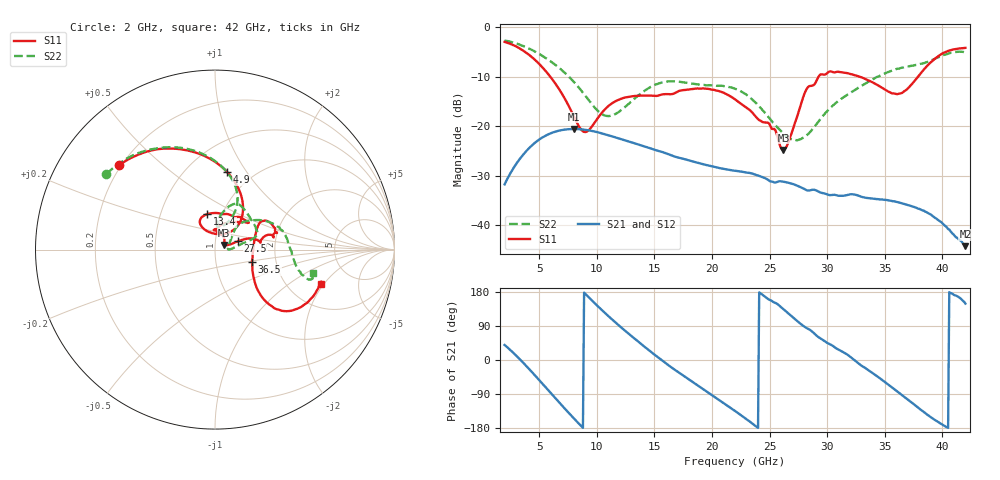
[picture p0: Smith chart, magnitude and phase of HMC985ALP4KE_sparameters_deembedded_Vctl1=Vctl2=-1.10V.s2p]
!s2p File: Measurements: S11, S21, S12, S22
# GHz S dB R 50.0
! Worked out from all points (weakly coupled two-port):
!   401 points, 2 GHz to 42 GHz, reference 50 ohm
!   highest |S21| = -20.57 dB at 8 GHz (marker M1); lowest = -44.3 dB at 42 GHz (marker M2)
!   lowest |S11| = -24.8 dB at 26.2 GHz (marker M3), VSWR 1.12, Z = 55.3 + j2.83 ohm
!   |S11| at or under -10 dB: 5.969 GHz to 29.25 GHz (23.28 GHz wide, 132 % of centre); 32.81 GHz to 37.88 GHz (5.074 GHz wide, 14.4 % of centre)
!   |S22| runs from -22.9 to -2.7 dB; largest |S21 - S12| = 0.00017
!   S11 on the Smith chart (normalised r, x): 2 GHz: 0.19, +0.36; 4.9 GHz: 0.76, +0.82; 13.4 GHz: 0.85, +0.35; 27.5 GHz: 1.29, +0.12; 36.5 GHz: 1.50, -0.21; 42 GHz: 3.02, -1.86
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2  -2.95 138.7  -31.79 39.7  -31.79 39.8  -2.65 145.2
3.4  -4.40 111.3  -26.39 -0.5  -26.39 -0.5  -3.59 122.4
4.9  -7.16 81.3  -22.88 -49.5  -22.89 -49.5  -5.24 99.0
6.3  -11.04 56.2  -21.19 -97.3  -21.20 -97.3  -7.41 79.6
8  -17.95 50.1  -20.57 -153.7  -20.58 -153.7  -11.01 64.0
8.7  -20.85 70.4  -20.66 -175.9  -20.66 -175.9  -12.94 62.2
10.9  -16.16 120.3  -21.76 118.8  -21.76 118.8  -17.95 79.9
13.4  -13.87 102.2  -23.56 53.3  -23.57 53.3  -14.18 80.6
15.4  -13.76 75.4  -25.05 5.3  -25.05 5.4  -11.33 68.5
18.9  -12.40 39.6  -27.50 -70.1  -27.50 -70.1  -11.59 41.5
22  -14.56 55.1  -29.03 -134.4  -29.03 -134.4  -12.42 17.8
24.9  -19.33 89.5  -30.92 160.4  -30.93 160.4  -18.14 8.9
26.2  -24.84 26.4  -31.24 133.8  -31.25 133.8  -21.50 0.9
27.5  -17.27 19.7  -32.15 100.1  -32.15 100.1  -22.76 6.1
28.2  -12.56 13.8  -32.95 84.5  -32.94 84.7  -21.91 18.1
28.7  -11.81 9.0  -32.89 75.0  -32.89 75.1  -20.67 26.5
31  -9.01 19.9  -34.09 27.3  -34.08 27.1  -14.83 46.7
33.3  -10.43 31.3  -34.48 -21.1  -34.50 -21.2  -11.42 37.5
35.4  -13.09 10.4  -35.05 -67.1  -35.06 -67.0  -8.97 23.6
36.5  -13.29 -18.2  -35.63 -92.7  -35.64 -92.9  -8.15 15.3
39.6  -5.93 -42.4  -38.95 -162.9  -38.88 -163.0  -6.12 -15.2
42  -4.16 -17.8  -44.29 148.8  -44.21 148.4  -5.03 -13.3
